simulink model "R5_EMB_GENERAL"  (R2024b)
settings: Solver=FixedStepDiscrete  StartTime=0.0  StopTime=S  FixedStep=T  RelTol=1e-3  EnableMultiTasking=on
undefined symbols (not defined in the file): Serial_Port, Standard_Devices, T
libraries: easyio x8, simulink x4

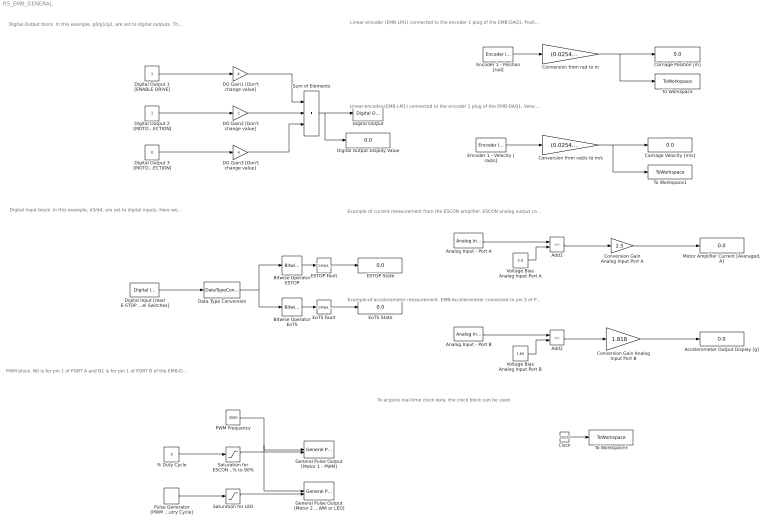
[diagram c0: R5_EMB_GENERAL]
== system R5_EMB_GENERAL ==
  note: Example of current measurement from the ESCON amplifier. ESCON analog output connected to pin 5 of PORT A (analog in).
  note: Example of accelerometer measurement. EMB-Accelerometer connected to pin 5 of PORT B (analog in).
  note: Linear encoder (EMB-LM1) connected to the encoder 1 plug of the EMB-DAQ1. Position reading with units in meters [m].
  note: Linear encoder (EMB-LM1) connected to the encoder 1 plug of the EMB-DAQ1. Velocity reading with units in meters/s [m/s]. For better measurements, consider using a high-pass filter on the position signal.
  note: Digital Output block. In this example, g0/g1/g2, are set to digital outputs. The gains are related to each output pin (gain =1 for g0, gain=2 for g1, gain=4 for g2) and the sum is fed to G0 block. Here we used constants, for inputs, but you can use signals such as the sign of a PID controller for motor direction.
  note: Digital Input block. In this example, d3/d4, are set to digital inputs. Here we used these digital inputs for a safety system. The E-STOP is d3 and the End-of-Travel Switch is d4 (EoTS). To isolate these states from the digital inputs, a Bitwise AND operation is performed. Since the Simulink Bitwise Operator accepts only integer data types, the signal is first converted to an unsigned 8-bit integer (uint8).
  note: PWM block. N0 is for pin 1 of PORT A and N1 is for pin 1 of PORT B of the EMB-DAQ1. We set the PWM mode to frequency and duty. The ESCON frequency range is from 10Hz to 5KHz and the duty is from 0.1 and 0.9%. N1 can be used to control another actuator or the the user LED of the EMB-DAQ1 (PORT B, pin 1 wired to LED).
  note: To acquire real-time clock data, the clock block can be used.
  % Duty Cycle : Constant  Value=0
  Accelerometer Output Display [g] : Display
  Add1 : Sum  Inputs=+-
  Add2 : Sum  Inputs=+-
  Analog Input - Port A : easyio/Analog Input  SampleTime=T  MaxMissedTicks=10  ShowMissedTicks=0  YieldWhenWaiting=0  DrvName=Standard_Devices/Serial_Port  DrvAddress=6  DrvOptions=[460800 8 0 0 0 0 0 0]  PacketSize=8  DataTypes='double'  ShowReady=0  ShowError=0  PacketID=1  ByteOrder=1  ShowTimestamp=0  CfgPrm=A6  PrmCfg=unipolar  ResVar=0  VarRes=0
  Analog Input - Port B : easyio/Analog Input  SampleTime=T  MaxMissedTicks=10  ShowMissedTicks=0  YieldWhenWaiting=0  DrvName=Standard_Devices/Serial_Port  DrvAddress=6  DrvOptions=[460800 8 0 0 0 0 0 0]  PacketSize=8  DataTypes='double'  ShowReady=0  ShowError=0  PacketID=1  ByteOrder=1  ShowTimestamp=0  CfgPrm=A7  PrmCfg=unipolar  ResVar=0  VarRes=0
  Bitwise Operator ESTOP : simulink/Logic and Bit Operations/Bitwise Operator  logicop=AND  UseBitMask=on  BitMask=8  BitMaskRealWorld=Real World Value
  Bitwise Operator EoTS : simulink/Logic and Bit Operations/Bitwise Operator  logicop=AND  UseBitMask=on  BitMask=16  BitMaskRealWorld=Real World Value
  Carriage Position [m] : Display
  Carriage Velocity [m/s] : Display
  Clock : Clock
  Conversion Gain Analog Input Port A : Gain  Gain=2.5
  Conversion Gain Analog Input Port B : Gain  Gain=1.818
  Conversion from rad to m : Gain  Gain=(0.0254)/(2*pi)
  Conversion from rad/s to m/s : Gain  Gain=(0.0254)/(2*pi)
  DO Gain1 [Don't change value] : Gain
  DO Gain2 [Don't change value] : Gain  Gain=2
  DO Gain3 [Don't change value] : Gain  Gain=4
  Data Type Conversion : DataTypeConversion  OutDataTypeStr=uint8  RndMeth=Nearest
  Digital Input [read E-STOP and End of Travel Switches] : easyio/Digital Input  SampleTime=T  MaxMissedTicks=10  ShowMissedTicks=0  YieldWhenWaiting=0  DrvName=Standard_Devices/Serial_Port  DrvAddress=6  DrvOptions=[460800 8 0 0 0 0 0 0]  PacketSize=8  DataTypes='double'  ShowReady=0  ShowError=0  PacketID=1  ByteOrder=1  ShowTimestamp=0  CfgPrm=D0  PrmCfg=18  ResVar=0  VarRes=0  d7=off  d6=off  d5=off  d4=on  d3=on  d2=off  d1=off  d0=off
  Digital Output : easyio/Digital Output  SampleTime=T  MaxMissedTicks=10  ShowMissedTicks=0  YieldWhenWaiting=0  DrvName=Standard_Devices/Serial_Port  DrvAddress=6  DrvOptions=[460800 8 0 0 0 0 0 0]  PacketSize=8  DataTypes='double'  ShowReady=0  ShowError=0  PacketID=1  ByteOrder=1  InitialValue=0  FinalValue=0  CfgPrm=G0  PrmCfg=F8  ResVar=0  VarRes=0  d7=off  d6=off  d5=off  d4=off  d3=off  d2=on  d1=on  d0=on
  Digital Output 1 [ENABLE DRIVE] : Constant
  Digital Output 2 [MOTOR 1 DIRECTION] : Constant
  Digital Output 3 [MOTOR 2 DIRECTION] : Constant  Value=0
  Digital Output Display Value : Display
  ESTOP Fault : simulink/Logic and Bit Operations/Compare To Constant  relop=~=  const=8  OutDataTypeStr=boolean
  ESTOP State : Display
  Encoder 1 - Position [rad] : easyio/Encoder Input  SampleTime=T  MaxMissedTicks=10  ShowMissedTicks=0  YieldWhenWaiting=0  DrvName=Standard_Devices/Serial_Port  DrvAddress=6  DrvOptions=[460800 8 0 0 0 0 0 0]  PacketSize=8  DataTypes='double'  ShowReady=0  ShowError=0  PacketID=1  ByteOrder=1  ShowTimestamp=0  CfgPrm=E0  PrmCfg=position  ResVar=0  VarRes=2000
  Encoder 1 - Velocity [ rad/s] : easyio/Encoder Input  SampleTime=T  MaxMissedTicks=10  ShowMissedTicks=0  YieldWhenWaiting=0  DrvName=Standard_Devices/Serial_Port  DrvAddress=6  DrvOptions=[460800 8 0 0 0 0 0 0]  PacketSize=8  DataTypes='double'  ShowReady=0  ShowError=0  PacketID=1  ByteOrder=1  ShowTimestamp=0  CfgPrm=E0  PrmCfg=velocity  ResVar=0  VarRes=2000
  EoTS Fault : simulink/Logic and Bit Operations/Compare To Constant  relop=~=  const=16  OutDataTypeStr=boolean
  EoTS State : Display
  General Pulse Output [Motor 1 - PWM] : easyio/General Pulse Output  SampleTime=T  MaxMissedTicks=10  ShowMissedTicks=0  YieldWhenWaiting=0  DrvName=Standard_Devices/Serial_Port  DrvAddress=6  DrvOptions=[460800 8 0 0 0 0 0 0]  PacketSize=16  DataTypes={'double','double'}  ShowReady=0  ShowError=0  PacketID=1  ByteOrder=1  InitialValue=[0 0]  FinalValue=[0 0]  CfgPrm=N0  PrmCfg=frequency and duty  ResVar=449.8360 Hz - 115156.25 Hz  VarRes=64
  General Pulse Output [Motor 2 - PWM or LED] : easyio/General Pulse Output  SampleTime=T  MaxMissedTicks=10  ShowMissedTicks=0  YieldWhenWaiting=0  DrvName=Standard_Devices/Serial_Port  DrvAddress=6  DrvOptions=[460800 8 0 0 0 0 0 0]  PacketSize=16  DataTypes={'double','double'}  ShowReady=0  ShowError=0  PacketID=1  ByteOrder=1  InitialValue=[0 0]  FinalValue=[0 0]  CfgPrm=N1  PrmCfg=frequency and duty  ResVar=449.8360 Hz - 115156.25 Hz  VarRes=64
  "Motor Amplifier Current [Averaged, A]" : Display
  PWM Frequency : Constant  Value=2000
  Pulse Generator [PWM % Dutry Cycle] : DiscretePulseGenerator  PulseType=Time based  Period=0.4  PulseWidth=50
  Saturation for ESCON 10% to 90% : Saturate  UpperLimit=0.9  LowerLimit=0.1
  Saturation for LED : Saturate  UpperLimit=1  LowerLimit=0
  Sum of Elements : Sum  Inputs=+++
  To Workspace : ToWorkspace  VariableName=position  SampleTime=-1
  To Workspace1 : ToWorkspace  VariableName=velocity  SampleTime=-1
  To Workspace3 : ToWorkspace  VariableName=rt_time  SampleTime=-1
  Voltage Bias Analog Input Port A : Constant  Value=2.0
  Voltage Bias Analog Input Port B : Constant  Value=1.65
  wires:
  Encoder 1 - Position [rad]/1 -> Conversion from rad to m/1
  PWM Frequency/1 -> General Pulse Output [Motor 1 - PWM]/1, General Pulse Output [Motor 2 - PWM or LED]/1
  Digital Output 1 [ENABLE DRIVE]/1 -> DO Gain1 [Don't change value]/1
  Sum of Elements/1 -> Digital Output/1, Digital Output Display Value/1
  DO Gain2 [Don't change value]/1 -> Sum of Elements/2
  DO Gain1 [Don't change value]/1 -> Sum of Elements/1
  Saturation for LED/1 -> General Pulse Output [Motor 2 - PWM or LED]/2
  Pulse Generator [PWM % Dutry Cycle]/1 -> Saturation for LED/1
  Digital Output 3 [MOTOR 2 DIRECTION]/1 -> DO Gain3 [Don't change value]/1
  DO Gain3 [Don't change value]/1 -> Sum of Elements/3
  Voltage Bias Analog Input Port A/1 -> Add1/2
  Analog Input - Port A/1 -> Add1/1
  Add1/1 -> Conversion Gain Analog Input Port A/1
  Voltage Bias Analog Input Port B/1 -> Add2/2
  Add2/1 -> Conversion Gain Analog Input Port B/1
  Analog Input - Port B/1 -> Add2/1
  Conversion Gain Analog Input Port B/1 -> Accelerometer Output Display [g]/1
  Conversion Gain Analog Input Port A/1 -> "Motor Amplifier Current [Averaged, A]"/1
  Conversion from rad to m/1 -> To Workspace/1, Carriage Position [m]/1
  Conversion from rad/s to m/s/1 -> To Workspace1/1, Carriage Velocity [m/s]/1
  Encoder 1 - Velocity [ rad/s]/1 -> Conversion from rad/s to m/s/1
  Clock/1 -> To Workspace3/1
  Digital Output 2 [MOTOR 1 DIRECTION]/1 -> DO Gain2 [Don't change value]/1
  % Duty Cycle/1 -> Saturation for ESCON 10% to 90%/1
  Saturation for ESCON 10% to 90%/1 -> General Pulse Output [Motor 1 - PWM]/2
  Bitwise Operator ESTOP/1 -> ESTOP Fault/1
  Bitwise Operator EoTS/1 -> EoTS Fault/1
  Data Type Conversion/1 -> Bitwise Operator ESTOP/1, Bitwise Operator EoTS/1
  Digital Input [read E-STOP and End of Travel Switches]/1 -> Data Type Conversion/1
  ESTOP Fault/1 -> ESTOP State/1
  EoTS Fault/1 -> EoTS State/1
